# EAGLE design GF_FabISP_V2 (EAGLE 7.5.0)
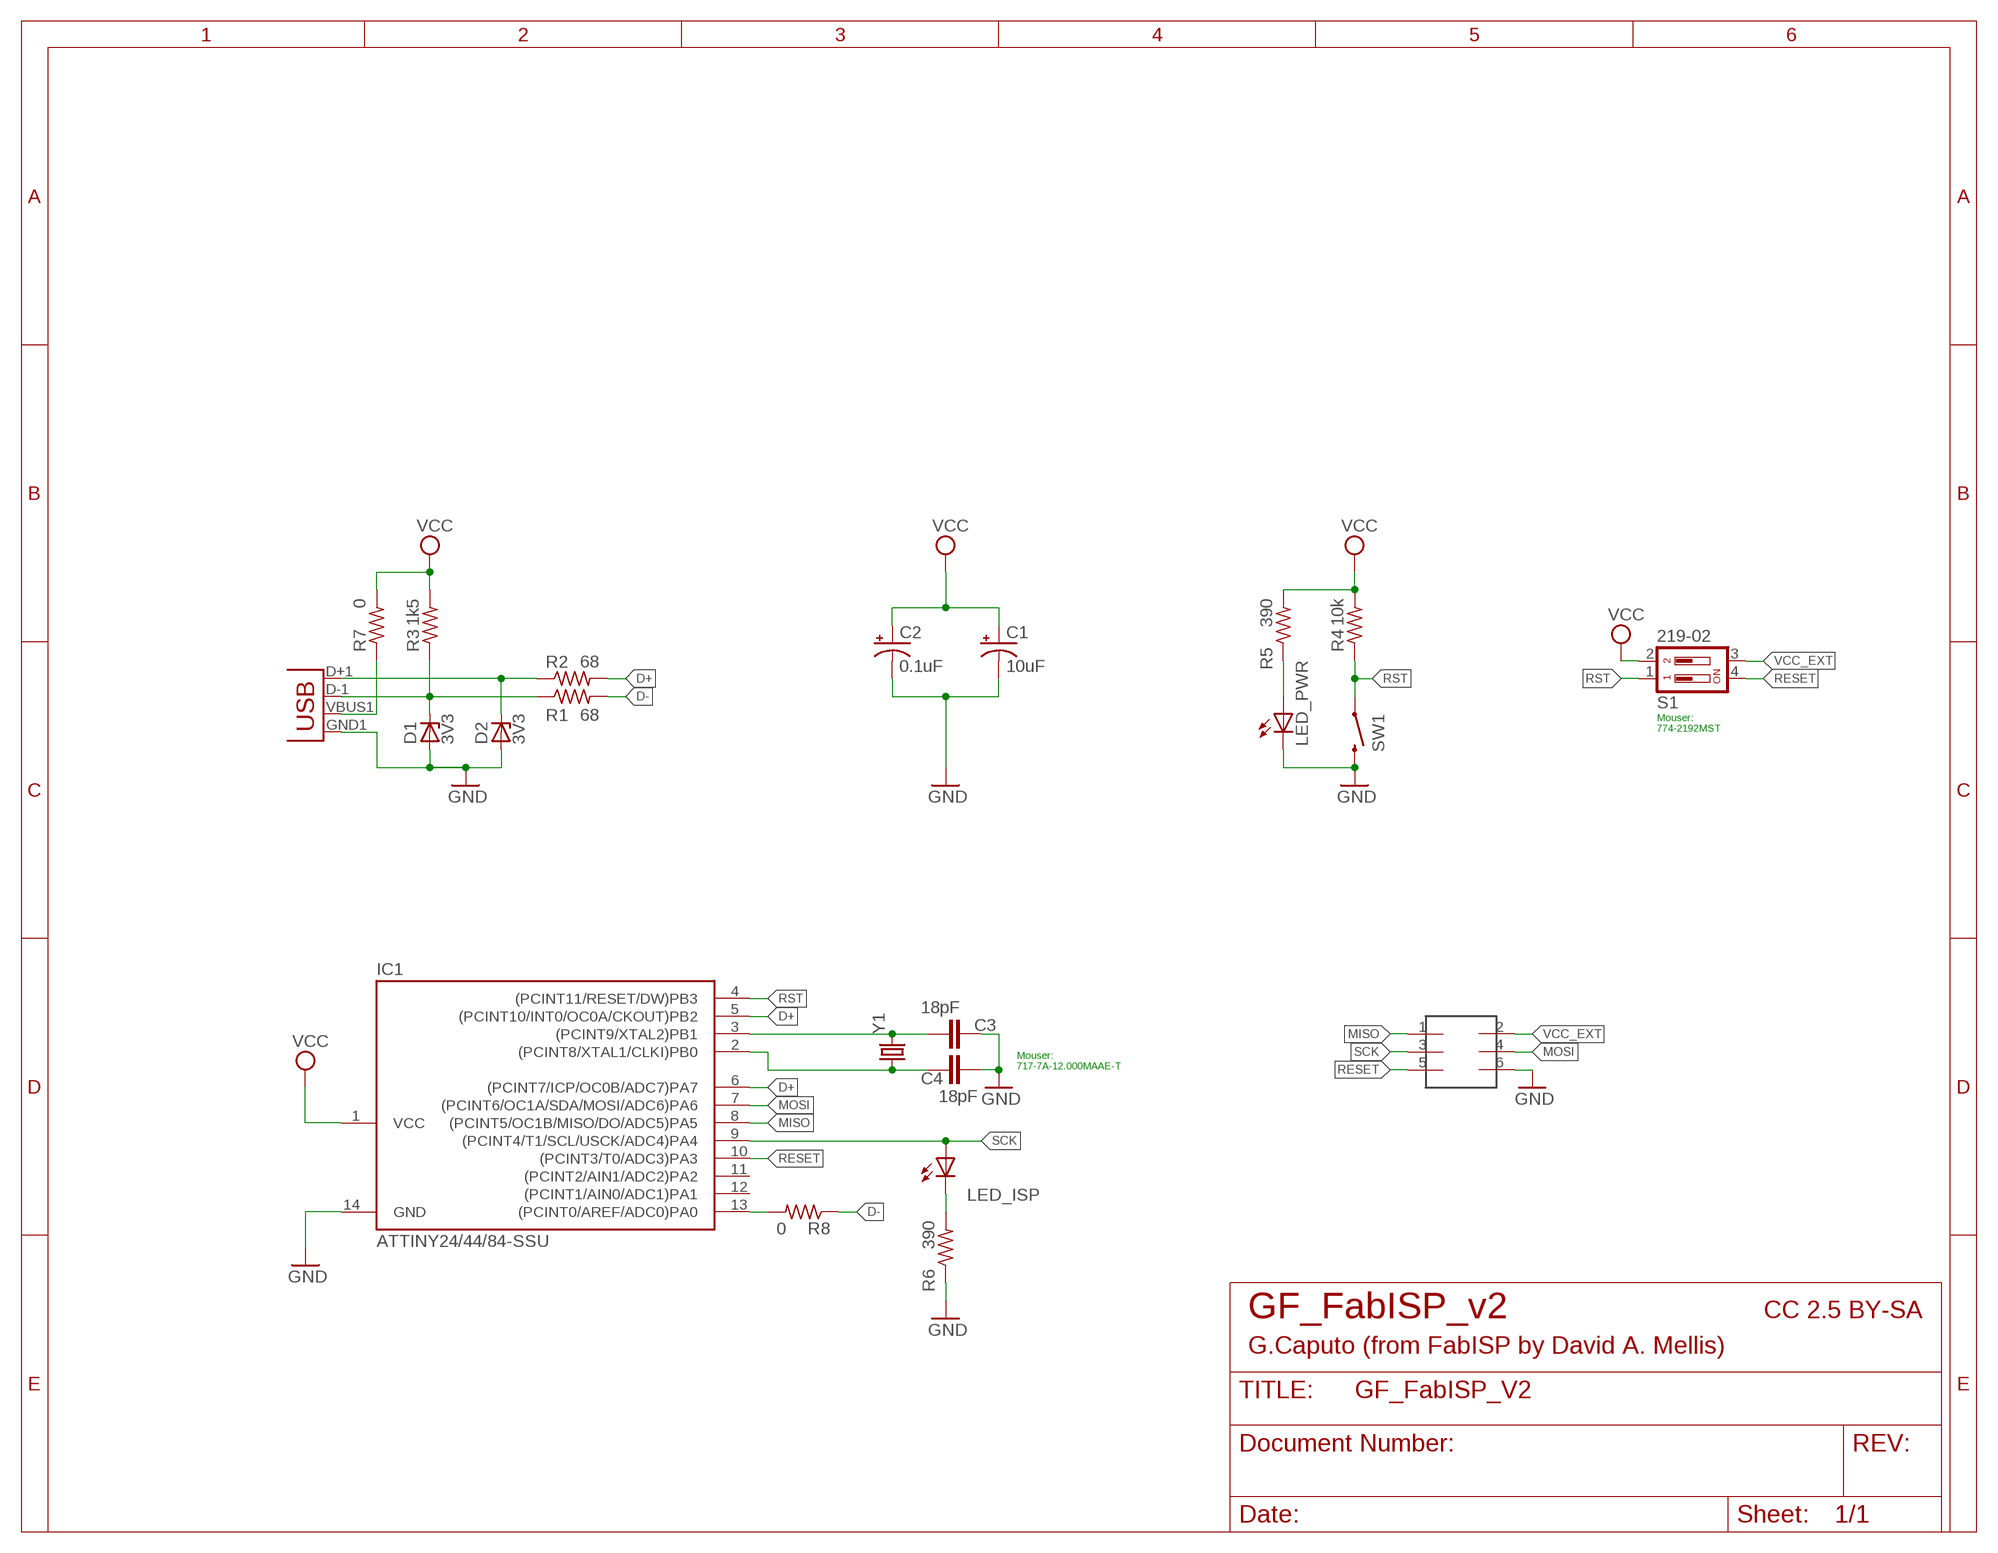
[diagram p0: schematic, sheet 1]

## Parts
C1  10uF  CPOL-USSMCA  [SMC_A]
C2  0.1uF  CPOL-USSMCA  [SMC_A]
C3  18pF  C-EUC0603K  [C0603K]
C4  18pF  C-EUC0603K  [C0603K]
D1  3V3  ZENER-DIODESOD80C  [SOD80C]
D2  3V3  ZENER-DIODESOD80C  [SOD80C]
IC1  ATTINY24/44/84-SSU  [SOIC14]
JP1  USBA-SMD-MALE  [USB-A-SMT-MALE]
LED_ISP  LEDCHIPLED_1206  [CHIPLED_1206]
LED_PWR  LEDCHIPLED_1206  [CHIPLED_1206]
R1  68  R-US_R1206  [R1206]
R2  68  R-US_R1206  [R1206]
R3  1k5  R-US_R1206  [R1206]
R4  10k  R-US_R1206  [R1206]
R5  390  R-US_R1206  [R1206]
R6  390  R-US_R0603  [R0603]
R7  0  R-US_R1206  [R1206]
R8  0  R-US_R1206  [R1206]
S1  219-02  [CTS-219-02]
SW1  SWITCH2  [TACTILE-SWITCH-1101NE]
U$1  2X3HEADER  [2X3_SMD]
Y1  CRYSTALTXC-7A  [CRYSTAL-TXC-7A]

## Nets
D+: IC1.5((PCINT10/INT0/OC0A/CKOUT)PB2) IC1.6((PCINT7/ICP/OC0B/ADC7)PA7) R2.2
D-: R1.2 R8.1
GND: C1.- C2.- C3.2 C4.2 D1.A D2.A IC1.14(GND) JP1.GND1(GND) LED_PWR.C R6.1 SW1.P$2 U$1.6
MISO: IC1.8((PCINT5/OC1B/MISO/DO/ADC5)PA5) U$1.1
MOSI: IC1.7((PCINT6/OC1A/SDA/MOSI/ADC6)PA6) U$1.4
N$1: D1.C JP1.D-1(D-) R1.1 R3.1
N$2: LED_PWR.A R5.1
N$3: D2.C JP1.D+1(D+) R2.1
N$4: LED_ISP.C R6.2
N$5: JP1.VBUS1(VBUS) R7.1
N$7: C3.1 IC1.3((PCINT9/XTAL2)PB1) Y1.P$2
N$8: C4.1 IC1.2((PCINT8/XTAL1/CLKI)PB0) Y1.P$1
N$9: IC1.13((PCINT0/AREF/ADC0)PA0) R8.2
RESET: IC1.10((PCINT3/T0/ADC3)PA3) S1.4 U$1.5
RST: IC1.4((PCINT11/RESET/DW)PB3) R4.1 S1.1 SW1.P$1
SCK: IC1.9((PCINT4/T1/SCL/USCK/ADC4)PA4) LED_ISP.A U$1.3
VCC: C1.+ C2.+ IC1.1(VCC) R3.2 R4.2 R5.2 R7.2 S1.2
VCC_EXT: S1.3 U$1.2
Unconnected: IC1.11((PCINT2/AIN1/ADC2)PA2) IC1.12((PCINT1/AIN0/ADC1)PA1)

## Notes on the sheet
- Mouser:
  774-2192MST
- Mouser:
  717-7A-12.000MAAE-T
- GF_FabISP_v2 | CC 2.5 BY-SA
- G.Caputo (from FabISP by David A. Mellis)

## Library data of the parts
C1 C2 = rcl:CPOL-US: POLARIZED CAPACITOR, American symbol
C3 C4 = rcl:C-EU: CAPACITOR, European symbol
D1 D2 = diode:ZENER-DIODE: Z-Diode
IC1 = attiny24_44_84:ATTINY24/44/84
JP1 = SparkFun-Connectors:USB: USB Connectors USB-B-PTH is fully proven SKU : PRT-00139/CONN-08278 USB-miniB is fully proven SKU : PRT-00587 USB-A-PCB is untested. USB-A-H is throughly reviewed, but untested. Spark Fun Electronics SKU : PRT-00437 USB-B-SMT is throughly reviewed, but untested. Needs silkscreen touching up.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
LED_ISP LED_PWR = led:LED: LED
R1-R8 = rcl:R-US_: RESISTOR, American symbol
S1 = switch-dil:219-02*: Surface Mount DIP Switch Series 219 SMT CTS Electronic Components Sourc: www.ctscorp.com; OC_FARNELL: unknown; OC_NEWARK: unknown
SW1 = SparkFun-Electromechanical:SWITCH2
U$1 = mellis:2X3HEADER
Y1 = SparkFun-FreqCtrl:CRYSTAL: Various standard crystals. Proven footprints. Spark Fun Electronics SKU : COM-00534

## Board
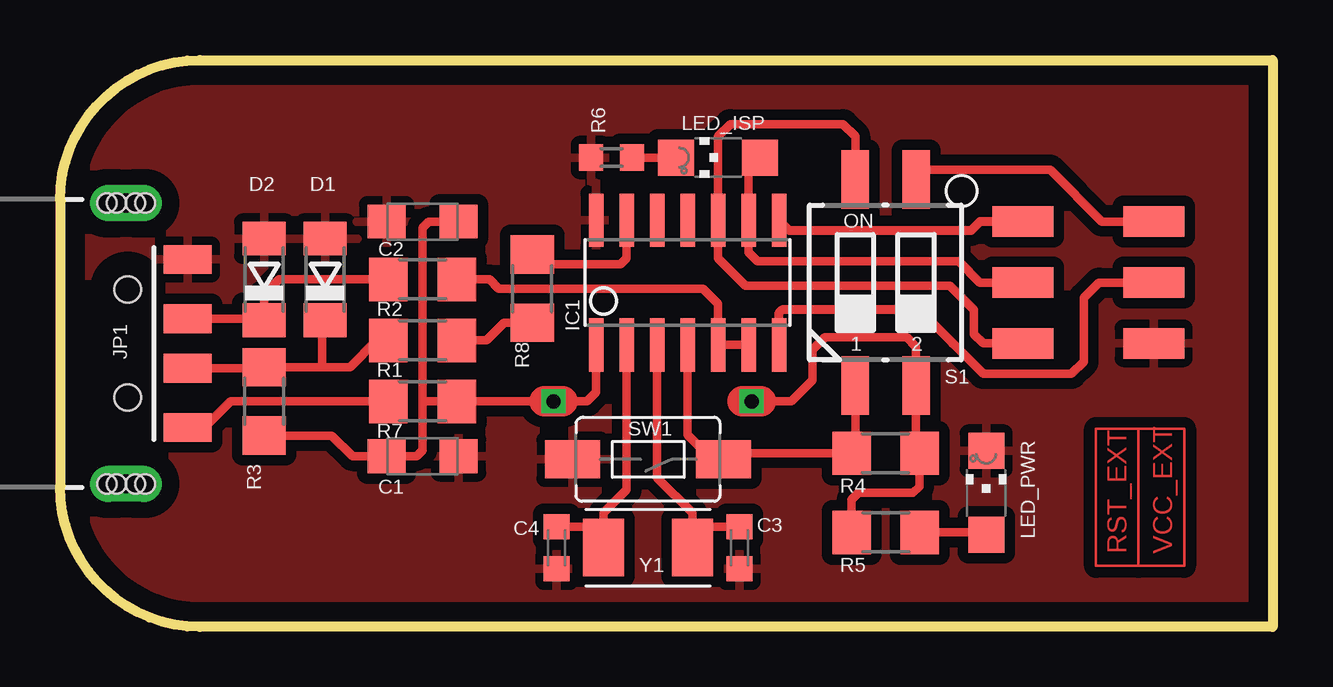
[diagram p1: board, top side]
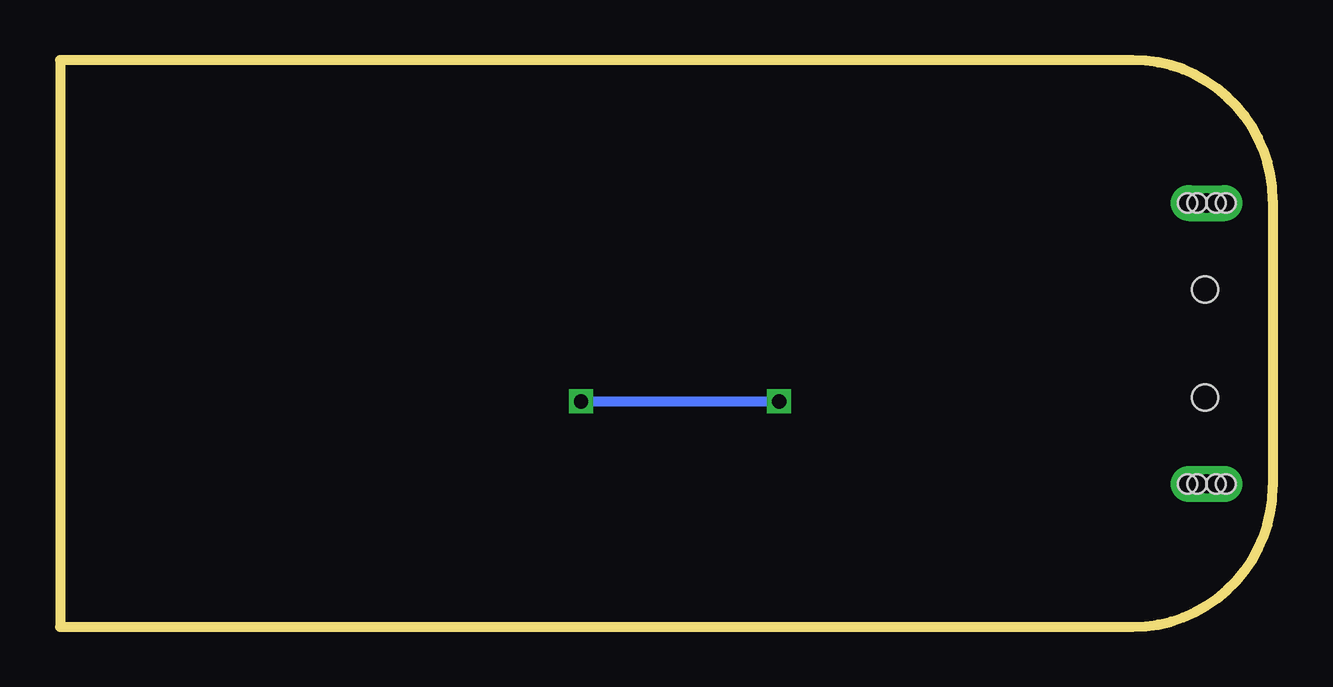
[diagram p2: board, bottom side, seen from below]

Size 50.55 x 23.62 mm. Coordinates in mm from the lower left corner, seen from the top.
Outline: 0,17.78 arc-90 5.84,23.62 50.55,23.62 50.55,0 5.84,0 arc-90 0,5.84 0,17.78
Copper layers (1*16): Top 0.035mm / dielectric 1.5mm / Bottom 0.035mm
Design rules "default *": minimum track width 10mil, minimum drill 24mil, track to track 16mil, track to pad 16mil, pad to pad 16mil, via to via 16mil, smd to smd 8mil, copper to edge 40mil, drill to drill 8mil, minimum pad ring 10mil, minimum via ring 8mil, stop-mask expansion 4mil, vias tented up to drill 0mil, thermal gap 0.35mm
Milling: 6 lines

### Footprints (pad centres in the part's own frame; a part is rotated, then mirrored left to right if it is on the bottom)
SMC_A = smd 1.6 x 1.4: + -1.5,0; - 1.5,0
C0603K = smd 1.05 x 1.08: 1 -0.875,0; 2 0.875,0
SOD80C = smd 1.4 x 1.8: A 1.7,0; C -1.7,0
SOIC14 = smd 0.61 x 2.21: 1 -3.81,-2.603; 2 -2.54,-2.603; 3 -1.27,-2.603; 4 0,-2.603; 5 1.27,-2.603; 6 2.54,-2.603; 7 3.81,-2.603; 8 3.81,2.603; 9 2.54,2.603; 10 1.27,2.603; 11 0,2.603; 12 -1.27,2.603; 13 -2.54,2.603; 14 -3.81,2.603
USB-A-SMT-MALE = smd 1.2 x 2: D+1 1.027,-3.67; D-1 -1.027,-3.67; GND1 3.5,-3.67; VBUS1 -3.5,-3.67 | drill 0.8 pad 1.5 long: P$1 5.85,-1.1; P$3 -5.85,-1.1 | hole 1.1: 2.25,-1.17; -2.25,-1.17 | hole 0.8: -5.85,-1.5; -5.85,-1.9; -5.85,-0.7; -5.85,-0.3; 5.85,-1.5; 5.85,-1.9; 5.85,-0.7; 5.85,-0.3
CHIPLED_1206 = smd 1.5 x 1.5: A 0,-1.75; C 0,1.75
R1206 = smd 1.6 x 1.803: 1 -1.422,0; 2 1.422,0
R0603 = smd 1 x 1.1: 1 -0.85,0; 2 0.85,0
CTS-219-02 = smd 1.13 x 2.44: 1 -1.27,-4.3; 2 1.27,-4.3; 3 1.27,4.3; 4 -1.27,4.3
TACTILE-SWITCH-1101NE = smd 2.3 x 1.6: P$1 -3.15,0; P$2 3.15,0
2X3_SMD = smd 2.54 x 1.27: 1 -2.54,2.54; 2 2.92,2.54; 3 -2.54,0; 4 2.92,0; 5 -2.54,-2.54; 6 2.92,-2.54
CRYSTAL-TXC-7A = smd 1.7 x 2.4: P$1 1.85,0; P$2 -1.85,0

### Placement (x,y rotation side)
C1  15.11,7.11 0 top
C2  15.11,16.89 180 top
C3  28.32,3.3 270 top
C4  20.7,3.3 270 top
D1  11.05,14.48 90 top
D2  8.51,14.48 90 top
IC1  26.16,14.35 0 top
JP1  1.65,11.81 90 top
LED_ISP  27.43,19.56 90 top
LED_PWR  38.61,5.59 0 top
R1  15.11,11.94 0 top
R2  15.11,14.48 0 top
R3  8.51,9.4 270 top
R4  34.42,7.24 0 top
R5  34.42,3.94 180 top
R6  22.99,19.56 0 top
R7  15.11,9.4 0 top
R8  19.68,14.1 90 top
S1  34.42,14.35 0 top
SW1  24.51,6.99 180 top
U$1  42.67,14.35 0 top
Y1  24.51,3.3 180 top

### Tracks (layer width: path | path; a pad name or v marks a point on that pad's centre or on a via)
D+
  Top 0.35: IC1.6 IC1.5 27.43,13.46 26.8,14.1 18.29,14.1 17.91,14.48 R2.2
D-
  Top 0.35: R8.1 18.52,12.68 17.78,11.94 R1.2
GND
  pour Top (isolate 0.45, rank 6): 0,0 50.55,0 50.55,23.62 0,23.62
MISO
  Top 0.38: U$1.1 38.35,16.89 37.97,16.51 30.42,16.51 IC1.8
MOSI
  Top 0.35: 37.21,11.81 38.48,10.54 42.16,10.54 42.67,11.05 42.67,13.72 43.31,14.35 U$1.4
  Top 0.38: IC1.7 29.97,13.08 30.1,13.21 35.81,13.21 37.21,11.81
N$1
  Top 0.35: JP1.D-1 8.51,10.78 R3.1 10.92,10.82 | 10.92,10.82 12.09,10.82 13.21,11.94 R1.1 | D1.C 10.92,12.65 10.92,10.82
N$2
  Top 0.35: R5.1 38.51,3.94 LED_PWR.A
N$3
  Top 0.35: JP1.D+1 8.51,12.84 | 8.51,12.84 D2.C | 8.51,12.84 8.51,13.84 9.14,14.48 R2.1
N$4
  Top 0.35: R6.2 LED_ISP.C
N$5
  Top 0.35: JP1.VBUS1 6.03,8.31 7.11,9.4 R7.1
N$6
  Top 0.1: 44.96,8.26 43.18,8.26 43.18,2.54 44.96,2.54 | 44.96,8.26 46.86,8.26 46.86,2.54 44.96,2.54 | 44.96,8.26 44.96,2.54
N$7
  Top 0.35: IC1.3 24.89,6.22 26.36,4.75 26.36,4.06 | Y1.P$2 26.36,4.06 | C3.1 26.47,4.18 26.36,4.06
N$8
  Top 0.35: IC1.2 23.62,5.71 22.66,4.75 22.66,3.81 | Y1.P$1 22.66,3.81 | C4.1 22.29,4.18 22.66,3.81
N$9
  Top 0.35: R8.2 20.09,15.11 23.37,15.11 23.62,15.37 IC1.13
RESET
  Top 0.35: S1.4 33.15,20.45 32.64,20.95 27.94,20.95 27.43,20.45 IC1.10 27.43,15.37 28.57,14.22 37.08,14.22 38.1,13.21 38.1,12.19 38.48,11.81 U$1.5
RST
  Top 0.35: IC1.4 26.16,8 26.8,7.37 27.28,7.37 SW1.P$1 27.91,7.24 R4.1 33.15,7.39 S1.1
SCK
  Top 0.35: LED_ISP.A 28.7,19.08 IC1.9 28.7,15.62 29.08,15.24 37.47,15.24 38.35,14.35 U$1.3
VCC  (via drill 0.6)
  Top 0.35: 8.17,8.31 R3.2 11.33,7.98 12.19,7.11 C1.+ 14.86,7.11 15.11,7.37 15.11,9.4 | 15.11,9.4 15.11,16.64 15.37,16.89 C2.+ | 15.11,9.4 R7.2 20.19,9.4 | R5.2 32.99,5.31 33.27,5.59 35.56,5.59 35.81,5.84 35.81,7.21 R4.2 35.69,7.39 S1.2 35.69,11.68 35.31,12.06 31.88,12.06 31.37,11.56 31.37,10.29 30.48,9.4 29.21,9.4 | 20.95,9.4 21.34,9.4 21.97,9.4 22.35,9.78 IC1.1
  Top 0.406: v20.57,9.4 21.34,9.4
  Top 1.27: 28.45,9.4 v28.83,9.4 29.21,9.4 | 20.19,9.4 v20.57,9.4 20.95,9.4
  Bottom 0.406: v28.83,9.4 v20.57,9.4
VCC_EXT
  Top 0.35: S1.3 36.09,19.05 41.27,19.05 43.43,16.89 U$1.2

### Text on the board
Top: RST_EXT | VCC_EXT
